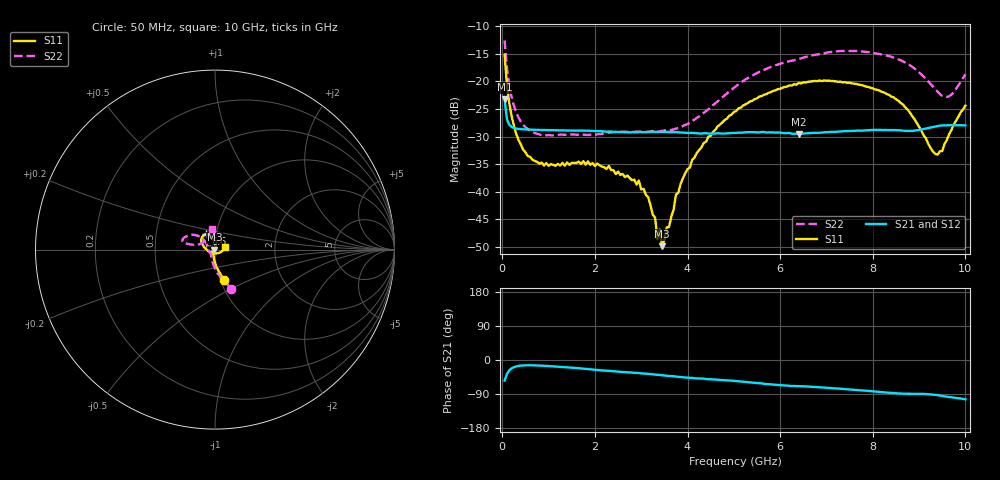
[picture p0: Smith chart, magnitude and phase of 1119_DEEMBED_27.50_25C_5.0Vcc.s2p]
!Hittite Microwave Corp.
!Digital Attenuator/PhaseShifter Rev 1.4.0
!Filename: C:\DATA\DATA\1119_DEEMBED_27.50_25C_5.0Vcc.s2p
!VNA ID: Agilent Technologies,N5224A,MY51441122,A.10.45.03
!Device type:
!2 Port Calibration.
!Temp(C): 25
!Lot Number:
!Serial Number:
!Operator:
!Misc:
!Attenuator:  27.500
# GHZ S DB R 50.0
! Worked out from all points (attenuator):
!   200 points, 50 MHz to 10 GHz, reference 50 ohm
!   highest |S21| = -23.26 dB at 50 MHz (marker M1); lowest = -29.5 dB at 6.4 GHz (marker M2)
!   lowest |S11| = -49.9 dB at 3.45 GHz (marker M3), VSWR 1.01, Z = 49.7 + j0.0548 ohm
!   |S11| at or under -10 dB: start of sweep to end of sweep
!   |S22| runs from -29.8 to -12.6 dB; largest |S21 - S12| = 0.00014
!   S11 on the Smith chart (normalised r, x): 50 MHz: 1.04, -0.36; 6.6 GHz: 0.89, +0.15; 10 GHz: 1.12, +0.03
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0.05  -15.14 -74.2  -23.26 -54.3  -23.26 -54.3  -12.56 -67.4
0.1  -20.61 -86.2  -26.86 -36.9  -26.86 -36.9  -17.51 -83.9
0.2  -26.25 -97.7  -28.24 -22.1  -28.27 -22.1  -22.78 -100.5
0.55  -33.55 -121.0  -28.74 -13.9  -28.75 -14.0  -28.66 -126.4
0.9  -35.27 -131.9  -28.82 -15.2  -28.82 -15.2  -29.76 -135.8
1.75  -34.47 -138.9  -28.93 -22.9  -28.93 -22.9  -29.66 -140.7
2.95  -37.99 -125.2  -29.18 -34.4  -29.19 -34.5  -29.13 -160.0
3.3  -44.71 -147.6  -29.16 -38.5  -29.17 -38.6  -29.05 -170.5
3.35  -48.67 -143.0  -29.17 -39.1  -29.18 -39.1  -29.09 -172.2
3.4  -46.86 -164.2  -29.16 -39.4  -29.17 -39.5  -29.03 -173.6
3.45  -49.90 170.1  -29.16 -40.1  -29.17 -40.2  -28.96 -175.4
3.75  -40.55 99.2  -29.20 -43.8  -29.21 -43.9  -28.57 173.2
4.1  -34.27 87.2  -29.33 -47.4  -29.33 -47.5  -27.18 158.3
5.05  -25.39 94.0  -29.33 -55.4  -29.34 -55.4  -20.83 138.7
6.4  -20.27 117.3  -29.51 -69.1  -29.52 -69.1  -15.93 149.9
6.6  -20.07 121.3  -29.41 -70.1  -29.41 -70.2  -15.46 152.8
6.7  -19.99 123.3  -29.34 -70.9  -29.35 -70.9  -15.25 153.9
8.35  -22.41 157.9  -28.83 -86.3  -28.83 -86.3  -15.41 168.1
8.75  -25.08 172.2  -28.97 -89.1  -28.97 -89.1  -16.78 168.1
9.400001  -33.28 -88.6  -28.09 -92.8  -28.11 -92.9  -21.86 153.7
9.65  -29.55 -27.0  -27.95 -97.5  -27.96 -97.6  -22.68 126.1
10  -24.41 13.8  -27.98 -103.7  -27.99 -103.7  -18.69 98.5
